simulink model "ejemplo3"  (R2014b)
settings: Solver=ode45  SolverMode=SingleTasking  StartTime=0.0  StopTime=8  RelTol=1e-6
libraries: simulink x3

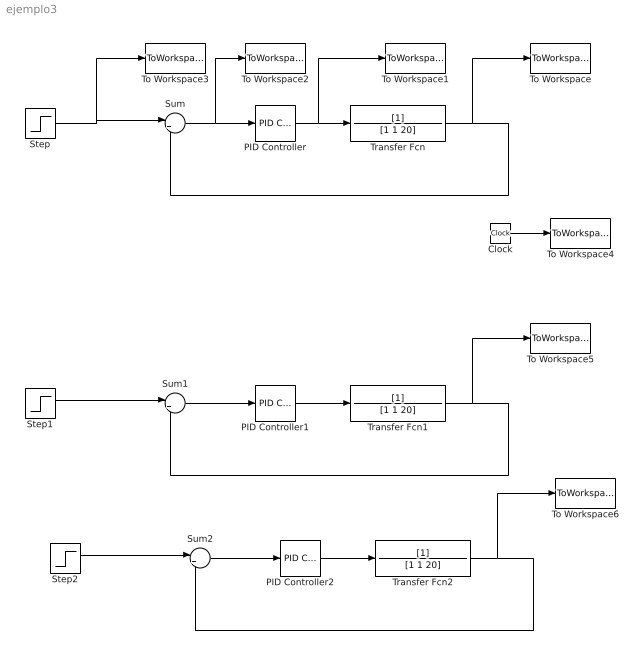
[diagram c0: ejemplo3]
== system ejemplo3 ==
  Clock : Clock
  PID Controller : simulink/Continuous/PID Controller  Controller=PID  TimeDomain=Continuous-time  SampleTime=-1  IntegratorMethod=Forward Euler  FilterMethod=Forward Euler  Form=Parallel  UseFilter=on  ControllerParametersSource=internal  P=42.641181646462  I=97.5167018870823  D=3.07629494754048  N=18.144758054021  InitialConditionSource=internal  InitialConditionForIntegrator=0  InitialConditionForFilter=0  ExternalReset=none  LimitOutput=off  UpperSaturationLimit=inf  LowerSaturationLimit=-inf  LinearizeAsGain=on  AntiWindupMode=none  Kb=1  TrackingMode=off  Kt=1  PParamMin=[]  PParamMax=[]  IParamMin=[]  IParamMax=[]  DParamMin=[]  DParamMax=[]  NParamMin=[]  NParamMax=[]  KbParamMin=[]  KbParamMax=[]  KtParamMin=[]  KtParamMax=[]  POutMin=[]  POutMax=[]  IOutMin=[]  IOutMax=[]  DOutMin=[]  DOutMax=[]  NOutMin=[]  NOutMax=[]  KbOutMin=[]  KbOutMax=[]  KtOutMin=[]  KtOutMax=[]  IntegratorOutMin=[]  IntegratorOutMax=[]  FilterOutMin=[]  FilterOutMax=[]  SumOutMin=[]  SumOutMax=[]  SumI1OutMin=[]  SumI1OutMax=[]  SumI2OutMin=[]  SumI2OutMax=[]  SumI3OutMin=[]  SumI3OutMax=[]  SumDOutMin=[]  SumDOutMax=[]  SaturationOutMin=[]  SaturationOutMax=[]  IntegratorContinuousStateAttributes=''  IntegratorStateMustResolveToSignalObject=off  IntegratorRTWStateStorageClass=Auto  FilterContinuousStateAttributes=''  FilterStateMustResolveToSignalObject=off  FilterRTWStateStorageClass=Auto  DifferentiatorICPrevScaledInput=0  DifferentiatorOutMin=[]  DifferentiatorOutMax=[]
  PID Controller1 : simulink/Continuous/PID Controller  Controller=PID  TimeDomain=Continuous-time  SampleTime=-1  IntegratorMethod=Forward Euler  FilterMethod=Forward Euler  Form=Parallel  UseFilter=on  ControllerParametersSource=internal  P=21.7880368510119  I=37.6526281244299  D=3.11850790777048  N=775.889322086618  InitialConditionSource=internal  InitialConditionForIntegrator=0  InitialConditionForFilter=0  ExternalReset=none  LimitOutput=off  UpperSaturationLimit=inf  LowerSaturationLimit=-inf  LinearizeAsGain=on  AntiWindupMode=none  Kb=1  TrackingMode=off  Kt=1  PParamMin=[]  PParamMax=[]  IParamMin=[]  IParamMax=[]  DParamMin=[]  DParamMax=[]  NParamMin=[]  NParamMax=[]  KbParamMin=[]  KbParamMax=[]  KtParamMin=[]  KtParamMax=[]  POutMin=[]  POutMax=[]  IOutMin=[]  IOutMax=[]  DOutMin=[]  DOutMax=[]  NOutMin=[]  NOutMax=[]  KbOutMin=[]  KbOutMax=[]  KtOutMin=[]  KtOutMax=[]  IntegratorOutMin=[]  IntegratorOutMax=[]  FilterOutMin=[]  FilterOutMax=[]  SumOutMin=[]  SumOutMax=[]  SumI1OutMin=[]  SumI1OutMax=[]  SumI2OutMin=[]  SumI2OutMax=[]  SumI3OutMin=[]  SumI3OutMax=[]  SumDOutMin=[]  SumDOutMax=[]  SaturationOutMin=[]  SaturationOutMax=[]  IntegratorContinuousStateAttributes=''  IntegratorStateMustResolveToSignalObject=off  IntegratorRTWStateStorageClass=Auto  FilterContinuousStateAttributes=''  FilterStateMustResolveToSignalObject=off  FilterRTWStateStorageClass=Auto  DifferentiatorICPrevScaledInput=0  DifferentiatorOutMin=[]  DifferentiatorOutMax=[]
  PID Controller2 : simulink/Continuous/PID Controller  Controller=PI  TimeDomain=Continuous-time  SampleTime=-1  IntegratorMethod=Forward Euler  FilterMethod=Forward Euler  Form=Parallel  UseFilter=on  ControllerParametersSource=internal  P=0  I=16.1280149525876  D=19.4141487866517  N=2453.5774699977  InitialConditionSource=internal  InitialConditionForIntegrator=0  InitialConditionForFilter=0  ExternalReset=none  LimitOutput=off  UpperSaturationLimit=inf  LowerSaturationLimit=-inf  LinearizeAsGain=on  AntiWindupMode=none  Kb=1  TrackingMode=off  Kt=1  PParamMin=[]  PParamMax=[]  IParamMin=[]  IParamMax=[]  DParamMin=[]  DParamMax=[]  NParamMin=[]  NParamMax=[]  KbParamMin=[]  KbParamMax=[]  KtParamMin=[]  KtParamMax=[]  POutMin=[]  POutMax=[]  IOutMin=[]  IOutMax=[]  DOutMin=[]  DOutMax=[]  NOutMin=[]  NOutMax=[]  KbOutMin=[]  KbOutMax=[]  KtOutMin=[]  KtOutMax=[]  IntegratorOutMin=[]  IntegratorOutMax=[]  FilterOutMin=[]  FilterOutMax=[]  SumOutMin=[]  SumOutMax=[]  SumI1OutMin=[]  SumI1OutMax=[]  SumI2OutMin=[]  SumI2OutMax=[]  SumI3OutMin=[]  SumI3OutMax=[]  SumDOutMin=[]  SumDOutMax=[]  SaturationOutMin=[]  SaturationOutMax=[]  IntegratorContinuousStateAttributes=''  IntegratorStateMustResolveToSignalObject=off  IntegratorRTWStateStorageClass=Auto  FilterContinuousStateAttributes=''  FilterStateMustResolveToSignalObject=off  FilterRTWStateStorageClass=Auto  DifferentiatorICPrevScaledInput=0  DifferentiatorOutMin=[]  DifferentiatorOutMax=[]
  Step : Step  SampleTime=0
  Step1 : Step  SampleTime=0
  Step2 : Step  SampleTime=0
  Sum : Sum  Inputs=|+-
  Sum1 : Sum  Inputs=|+-
  Sum2 : Sum  Inputs=|+-
  To Workspace : ToWorkspace  VariableName=salida  SampleTime=-1
  To Workspace1 : ToWorkspace  VariableName=entrada  SampleTime=-1
  To Workspace2 : ToWorkspace  VariableName=error1  SampleTime=-1
  To Workspace3 : ToWorkspace  VariableName=referencia  SampleTime=-1
  To Workspace4 : ToWorkspace  VariableName=tiempo  SampleTime=-1
  To Workspace5 : ToWorkspace  VariableName=salida2  SampleTime=-1
  To Workspace6 : ToWorkspace  VariableName=salida3  SampleTime=-1
  Transfer Fcn : TransferFcn  Denominator=[1 1 20]
  Transfer Fcn1 : TransferFcn  Denominator=[1 1 20]
  Transfer Fcn2 : TransferFcn  Denominator=[1 1 20]
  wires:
  PID Controller/1 -> To Workspace1/1, Transfer Fcn/1
  Step/1 -> To Workspace3/1, Sum/1
  Sum/1 -> To Workspace2/1, PID Controller/1
  Transfer Fcn/1 -> To Workspace/1, Sum/2
  Clock/1 -> To Workspace4/1
  Transfer Fcn1/1 -> Sum1/2, To Workspace5/1
  Sum1/1 -> PID Controller1/1
  Step1/1 -> Sum1/1
  PID Controller1/1 -> Transfer Fcn1/1
  PID Controller2/1 -> Transfer Fcn2/1
  Step2/1 -> Sum2/1
  Sum2/1 -> PID Controller2/1
  Transfer Fcn2/1 -> To Workspace6/1, Sum2/2
